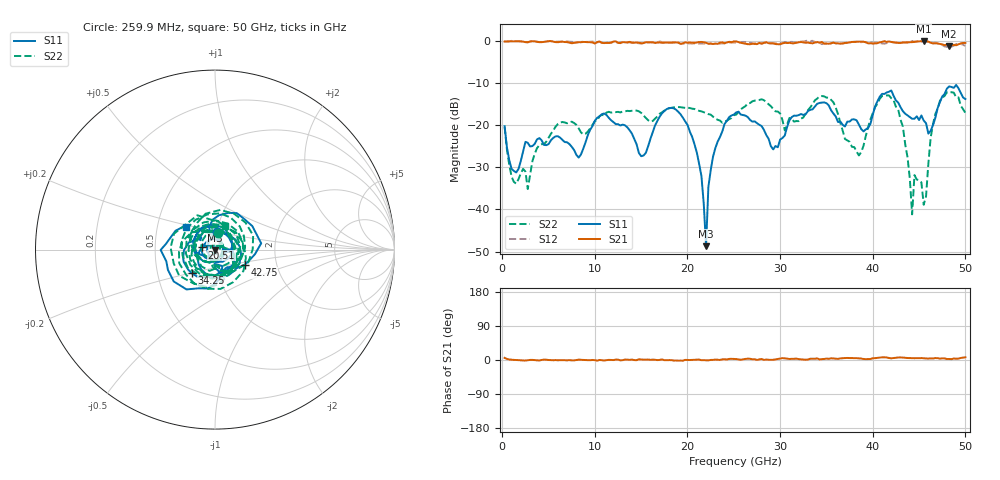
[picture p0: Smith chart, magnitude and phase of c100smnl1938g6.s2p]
! 5/12/2023 4:41:43 PM
! D:\C100SMNL1938G6.S2P
! CHANNEL.1
! TR.MEASUREMENT
! CORRECTED.DATA
# GHZ S RI R 50.0
! FREQ.GHZ  S11RE  S11IM  S21RE  S21IM  S12RE  S12IM  S22RE  S22IM
!; PortSelection: Port_12
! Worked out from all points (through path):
!   200 points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, 259.9 MHz to 50 GHz, reference 50 ohm
!   highest |S21| = 0.04 dB at 45.5 GHz (marker M1); lowest = -1.1 dB at 48.25 GHz (marker M2)
!   lowest |S11| = -48.7 dB at 22.01 GHz (marker M3), VSWR 1.01, Z = 49.9 - j0.363 ohm
!   |S11| at or under -10 dB: start of sweep to end of sweep
!   |S22| runs from -41.2 to -12.1 dB; largest |S21 - S12| = 0.094
!   S11 on the Smith chart (normalised r, x): 259.9 MHz: 1.01, +0.20; 20.51 GHz: 0.87, +0.02; 34.25 GHz: 0.75, -0.20; 42.75 GHz: 1.37, -0.24; 50 GHz: 0.70, +0.19
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0.25995  0.0132 0.0968  0.9862 0.0964  0.9866 0.0915  0.016 0.0947
1.25975  0.0245 0.0149  0.9954 0.00437  1.001 0.0143  0.013 -0.0168
2.75945  0.0549 -0.0288  0.9728 -0.00839  0.9673 -0.00559  0.00373 0.0171
6.0088  -0.0737 -0.00881  0.9723 -0.0115  0.9875 -0.0105  -0.0143 0.1028
8.75825  0.0192 -0.0495  0.9793 -0.00247  0.9856 0.00615  -0.0253 -0.0738
17.0066  0.1149 0.055  0.9669 0.00426  0.9942 0.0156  0.1061 -0.0873
20.5059  -0.072 0.0118  0.958 0.00275  0.9356 0.0103  0.1562 -0.0226
22.0056  -0.000494 -0.00363  0.9574 -0.0104  0.9344 0.00126  -0.0896 -0.1073
22.75545  -0.0262 -0.0332  0.9267 0.0048  0.9256 -9.28e-05  -0.1264 0.00931
25.25495  -0.0753 0.1207  0.9945 0.0439  0.9554 0.00982  0.129 -0.0362
29.25415  0.0517 -0.00312  0.9416 0.00947  0.9506 0.0115  0.1552 -0.0196
33.5033  -0.0408 -0.1494  0.9418 0.0548  1.011 0.0366  0.1722 -0.047
34.25315  -0.1294 -0.1314  0.96 0.0263  0.9588 0.0534  0.0313 -0.2189
38.5023  -0.0247 0.0992  0.9851 0.0767  0.9739 0.0752  0.0433 0.00691
41.75165  0.242 0.0655  0.9889 0.0924  0.9683 0.1259  0.2125 0.0792
42.75145  0.1657 -0.0842  0.9479 0.109  0.9654 0.0905  0.0816 -0.13
44.25115  0.0692 -0.0977  0.9705 0.0805  1.001 0.106  0.0007 -0.00872
44.5011  0.0571 -0.1054  0.9793 0.0796  0.9848 0.1064  0.00832 -0.0242
45.5009  0.0138 -0.1131  1.002 0.0797  0.9738 0.0821  -0.00538 -0.01
46.75065  0.0392 -0.1157  0.9414 0.083  0.961 0.0584  0.1017 -0.0907
48.25035  -0.2298 -0.1775  0.8786 0.0415  0.8595 0.0847  -0.23 -0.0773
50  -0.1618 0.1265  0.9475 0.1201  0.8739 0.0936  0.055 0.1288
